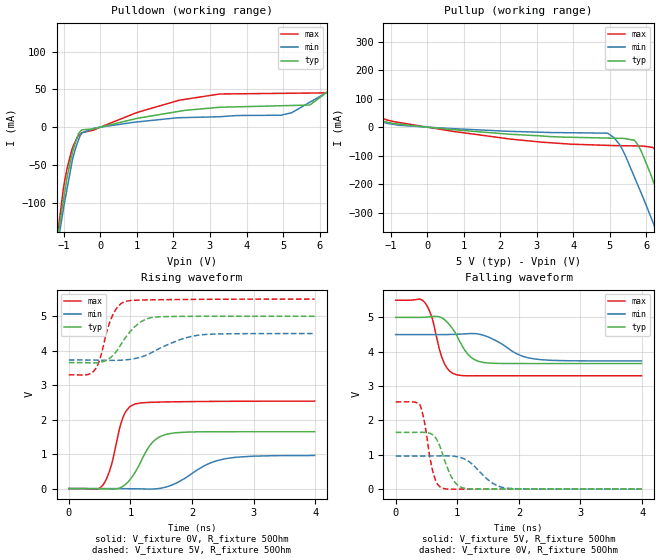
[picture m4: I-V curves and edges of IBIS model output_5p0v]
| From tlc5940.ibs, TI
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|   output_5p0v Model
[Model]   output_5p0v
Model_type   Output
Polarity   Non-Inverting
Vmeas = 2.5
Vref = 2.5
Cref = 15pF
Rref = 50
|   typ   min   max
|   (nom PVT)   (Fast PVT)   (slow PVT)
|Average
C_comp   1.546e-12   1.528e-12   1.582e-12
|ON state : BUFFER OUTPUT TURNED HIGH
|C_comp   1.624e-12   1.602e-12   1.689e-12
|OFF state: BUFFER is in LOW state
|C_comp   1.468e-12   1.454e-12   1.474e-12
| Where nom  PVT is Nominal Process, 5V, 65C
|   Fast PVT is Strong Process,  5.5V, -40C
|   Slow PVT is Weak Process,   4.5V, 125C
[Voltage Range]   5   4.5   5.5
|Ambient Temperature   25   85   -40
|Junction Temperature
[Temperature Range]   65   125   -40
[Pullup Reference]   5   4.5   5.5
[Pulldown Reference]   0   0   0
[Power Clamp Reference]   5   4.5   5.5
[GND Clamp Reference]   0   0   0
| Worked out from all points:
|   slope of the pulldown table from 0 to 0.75 V, typ, clamps not added: 86.1 ohm
|   slope of the pullup table from 0 to 0.75 V, typ, clamps not added: 80.7 ohm
|   falling waveform, V_fixture 5V, R_fixture 50Ohm: 20-80 % time 277ps typ, 435ps min, 195ps max; typ from 5 V to 3.66 V
|   rising waveform, V_fixture 0V, R_fixture 50Ohm: 20-80 % time 325ps typ, 558ps min, 212ps max; typ from 0 V to 1.65 V
|   rising waveform, V_fixture 5V, R_fixture 50Ohm: 20-80 % time 347ps typ, 577ps min, 218ps max; typ from 3.65 V to 5 V
|   falling waveform, V_fixture 0V, R_fixture 50Ohm: 20-80 % time 213ps typ, 345ps min, 146ps max; typ from 1.65 V to 0 V
[Pulldown]
|   Voltage   I(typ)   I(min)   I(max)
-5V       -1.613A    -1.455A    -1.865A
-1.145V   -138.6mA   -148.2mA   -131.9mA
-913.5mV  -67.57mA   -82.29mA   -55.13mA
-761mV    -33.53mA   -42.53mA   -27.41mA
-506.5mV  -3.567mA   -7.641mA   -7.401mA
2.167V    21.1mA     12.49mA    35.75mA
5.233V    28.73mA    19.06mA    44.96mA
5.74V     29.56mA    33.22mA    45.22mA
6.473V    58.51mA    53.76mA    51.67mA
7.789V    117.1mA    93mA       167.5mA
9.13V     181.9mA    135.9mA    293.8mA
10V       224.3mA    164.5mA    381.6mA
[Pullup]
|   Voltage   I(typ)   I(min)   I(max)
-5V       186.1mA    126.8mA    362.9mA
-1.117V   18.04mA    14.06mA    25.56mA
2.271V    -25mA      -14.82mA   -41.8mA
4.936V    -38.37mA   -21.12mA   -63.99mA
5.264V    -39.28mA   -61.06mA   -65.03mA
5.67V     -45.91mA   -174.8mA   -65.89mA
6.258V    -214.8mA   -359.8mA   -80.78mA
6.473V    -289.6mA   -429.1mA   -122.6mA
6.671V    -361.2mA   -494.7mA   -193.8mA
6.955V    -465.5mA   -590.4mA   -318.9mA
7.195V    -555.6mA   -671.6mA   -424.2mA
10V       -1.658A    -1.657A    -1.702A
[Ramp]
R_load = 50
|   typ   min   max
dV/dt_r   0.990395/3.24278e-10   0.576461/5.56559e-10   1.52268/2.1185e-10
dV/dt_f   0.806697/2.76446e-10   0.461463/4.34868e-10   1.31992/1.94528e-10
[Falling Waveform]
V_fixture = 5V
V_fixture_min = 4.5V
V_fixture_max = 5.5V
R_fixture = 50Ohm
|   Time   V(typ)   V(min)   V(max)
0s        5V         4.5V       5.5V
470ps     5.004V     4.5V       5.438V
590ps     5.024V     4.5V       4.988V
700ps     5.021V     4.499V     4.14V
780ps     4.948V     4.5V       3.699V
980ps     4.508V     4.508V     3.335V
1.19ns    3.893V     4.528V     3.299V
1.42ns    3.689V     4.482V     3.3V
2.23ns    3.656V     3.796V     3.3V
3.99ns    3.656V     3.731V     3.3V
[Rising Waveform]
V_fixture = 0V
V_fixture_min = 0V
V_fixture_max = 0V
R_fixture = 50Ohm
|   Time   V(typ)   V(min)   V(max)
0s        305.8pV    1.76nV     264.4pV
460ps     -1.869mV   538uV      -16.8mV
550ps     -5.626mV   732.2uV    95.58mV
690ps     -16.16mV   280.2uV    676.5mV
880ps     67.9mV     -2.029mV   2.067V
1.07ns    454mV      -5.618mV   2.448V
1.34ns    1.304V     -13.49mV   2.504V
1.6ns     1.581V     57mV       2.515V
2.5ns     1.65V      850.7mV    2.532V
3.99ns    1.651V     960.8mV    2.538V
[Rising Waveform]
V_fixture = 5V
V_fixture_min = 4.5V
V_fixture_max = 5.5V
R_fixture = 50Ohm
|   Time   V(typ)   V(min)   V(max)
0s        3.655V     3.731V     3.3V
420ps     3.647V     3.729V     3.442V
500ps     3.661V     3.726V     3.735V
620ps     3.731V     3.721V     4.573V
710ps     3.853V     3.719V     5.025V
920ps     4.38V      3.734V     5.431V
1.17ns    4.836V     3.815V     5.471V
1.42ns    4.978V     4.017V     5.479V
2.16ns    4.999V     4.464V     5.491V
3.99ns    5V         4.5V       5.499V
[Falling Waveform]
V_fixture = 0V
V_fixture_min = 0V
V_fixture_max = 0V
R_fixture = 50Ohm
|   Time   V(typ)   V(min)   V(max)
0s        1.651V     961.7mV    2.539V
390ps     1.654V     961.7mV    2.461V
460ps     1.652V     962.2mV    2.014V
610ps     1.576V     964.1mV    462.9mV
770ps     967.4mV    967.1mV    21.36mV
950ps     223.5mV    955.4mV    -2.005mV
1.15ns    13.2mV     845.7mV    146.5uV
1.56ns    428.6uV    189.2mV    321.8uV
1.79ns    210uV      29.85mV    322.2uV
3.99ns    135.1uV    61.4uV     285.6uV
